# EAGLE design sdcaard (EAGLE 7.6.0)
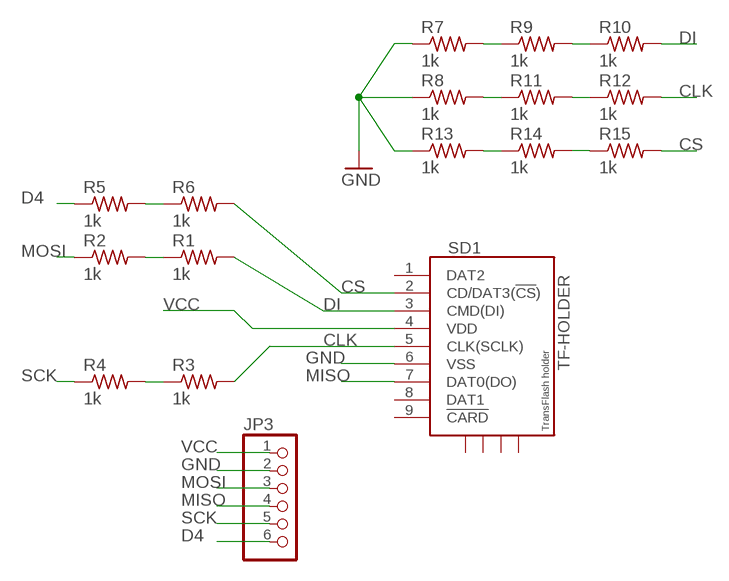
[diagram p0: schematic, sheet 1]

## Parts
JP3  PINHD-1X6  [1X06]
R1  1k  RES-US1206FAB  [R1206FAB]
R2  1k  RES-US1206FAB  [R1206FAB]
R3  1k  RES-US1206FAB  [R1206FAB]
R4  1k  RES-US1206FAB  [R1206FAB]
R5  1k  RES-US1206FAB  [R1206FAB]
R6  1k  RES-US1206FAB  [R1206FAB]
R7  1k  RES-US1206FAB  [R1206FAB]
R8  1k  RES-US1206FAB  [R1206FAB]
R9  1k  RES-US1206FAB  [R1206FAB]
R10  1k  RES-US1206FAB  [R1206FAB]
R11  1k  RES-US1206FAB  [R1206FAB]
R12  1k  RES-US1206FAB  [R1206FAB]
R13  1k  RES-US1206FAB  [R1206FAB]
R14  1k  RES-US1206FAB  [R1206FAB]
R15  1k  RES-US1206FAB  [R1206FAB]
SD1  TF-HOLDER  [TF-PULL]

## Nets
CLK: R3.2 R12.2 SD1.5(CLK(SCLK))
CS: R6.2 R15.2 SD1.2(CD/DAT3(!CS!))
D4: JP3.6 R5.1
DI: R1.2 R10.2 SD1.3(CMD(DI))
GND: JP3.2 R7.1 R8.1 R13.1 SD1.6(VSS)
MISO: JP3.4 SD1.7(DAT0(DO))
MOSI: JP3.3 R2.1
N$5: R1.1 R2.2
N$6: R5.2 R6.1
N$7: R3.1 R4.2
N$8: R13.2 R14.1
N$9: R14.2 R15.1
N$10: R8.2 R11.1
N$11: R7.2 R9.1
N$12: R9.2 R10.1
N$13: R11.2 R12.1
SCK: JP3.5 R4.1
VCC: JP3.1 SD1.4(VDD)
Unconnected: SD1.1(DAT2) SD1.8(DAT1) SD1.9(!CARD) SD1.S1 SD1.S2 SD1.S3 SD1.S4

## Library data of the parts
JP3 = pinhead:PINHD-1X6: PIN HEADER
R1-R15 = fab:RES-US: Resistor (US Symbol)
SD1 = sd-mmc:TF-HOLDER: TF / Micro SD socket is PUSH-PUSH type, the card can be pushed into and auto locked and pushed out by simply press the card. Surface Mounting type.

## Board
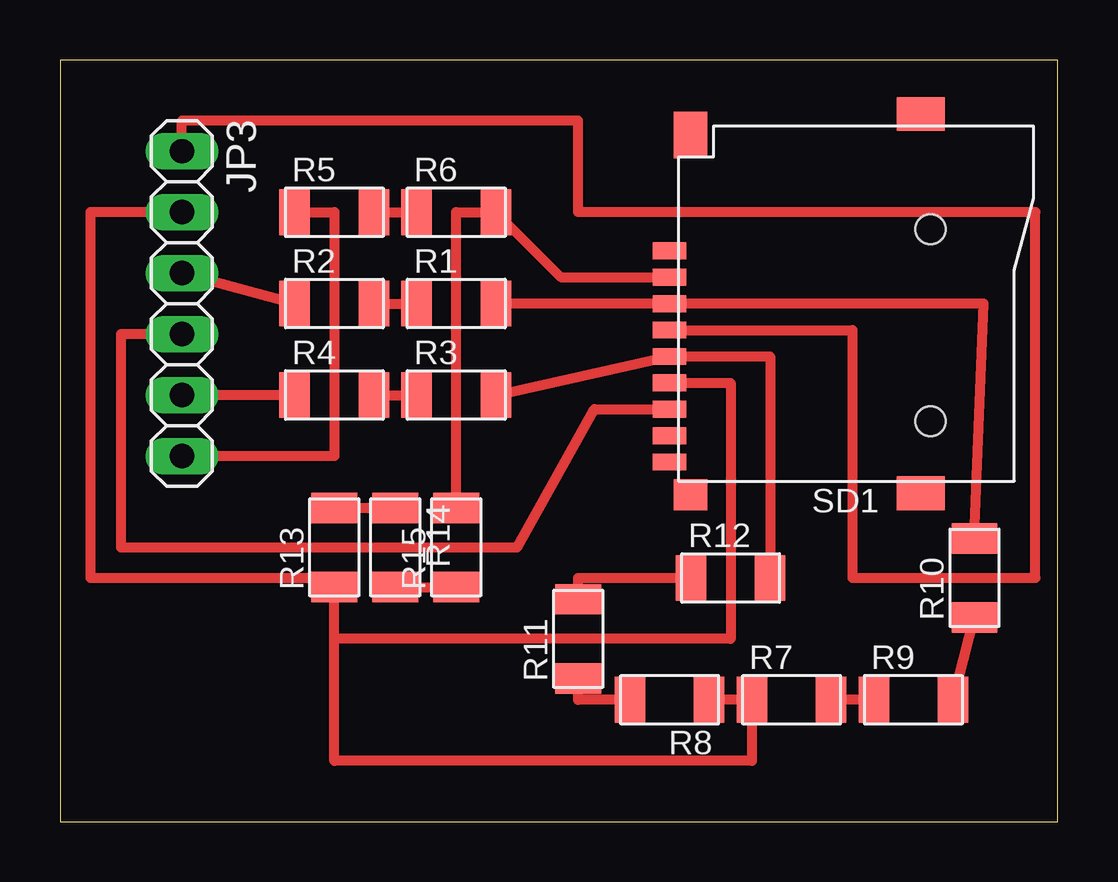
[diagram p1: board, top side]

Size 41.58 x 31.74 mm. Coordinates in mm from the lower left corner, seen from the top.
Outline: 0,0 41.58,0 41.58,31.74 0,31.74 0,0
Copper layers (1*16): Top 0.035mm / dielectric 1.5mm / Bottom 0.035mm
Design rules "default": minimum track width 10mil, minimum drill 24mil, track to track 8mil, track to pad 8mil, pad to pad 8mil, via to via 8mil, smd to smd 8mil, copper to edge 40mil, drill to drill 8mil, minimum pad ring 10mil, minimum via ring 8mil, stop-mask expansion 4mil, vias tented up to drill 0mil, thermal gap 10mil

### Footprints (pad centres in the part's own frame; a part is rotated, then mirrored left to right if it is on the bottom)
1X06 = drill 1.016 long: 1 -6.35,0; 2 -3.81,0; 3 -1.27,0; 4 1.27,0; 5 3.81,0; 6 6.35,0
R1206FAB = smd 1.27 x 1.905: 1 -1.651,0; 2 1.651,0
TF-PULL = smd 0.7 x 1.4: 1 -2.2,-7.62; 2 -1.1,-7.62; 3 0,-7.62; 4 1.1,-7.62; 5 2.2,-7.62; 6 3.3,-7.62; 7 4.4,-7.62; 8 5.5,-7.62; 9 6.6,-7.62 | smd 1.4 x 2: S1 -7.9,2.85; S2 7.9,2.85 | smd 1.28 x 1.4: S3 7.96,-6.75 | smd 1.95 x 1.4: S4 -7.025,-6.75 | hole 1.25: -3.1,3.25; 4.9,3.25

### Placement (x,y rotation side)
JP3  5.08,21.59 270 top
R1  16.51,21.59 0 top
R2  11.43,21.59 0 top
R3  16.51,17.78 0 top
R4  11.43,17.78 0 top
R5  11.43,25.4 0 top
R6  16.51,25.4 0 top
R7  30.48,5.08 0 top
R8  25.4,5.08 180 top
R9  35.56,5.08 0 top
R10  38.1,10.16 90 top
R11  21.59,7.62 90 top
R12  27.94,10.16 0 top
R13  11.43,11.43 90 top
R14  13.97,11.43 270 top
R15  16.51,11.43 90 top
SD1  33.02,21.59 270 top

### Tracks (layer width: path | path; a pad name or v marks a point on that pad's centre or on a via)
CLK
  Top 0.406: R3.2 SD1.5 29.59,19.39 R12.2
CS
  Top 0.406: SD1.2 20.87,22.69 R6.2 16.51,25.4 R15.2
D4
  Top 0.406: R5.1 11.43,25.4 11.43,15.24 JP3.6
DI
  Top 0.406: R1.2 SD1.3 38.48,21.59 R10.2
GND
  Top 0.406: JP3.2 1.27,25.4 1.27,10.16 11.43,10.16 R13.1 | R8.1 R7.1 28.83,2.54 11.43,2.54 R13.1 | SD1.6 27.94,18.29 27.94,7.62 11.43,7.62 R13.1
MISO
  Top 0.406: JP3.4 2.54,20.32 2.54,11.43 19.05,11.43 22.27,17.19 SD1.7
MOSI
  Top 0.406: R2.1 JP3.3
N$5
  Top 0.406: R2.2 R1.1
N$6
  Top 0.406: R5.2 R6.1
N$7
  Top 0.406: R4.2 R3.1
N$8
  Top 0.406: R13.2 R14.1
N$9
  Top 0.406: R14.2 R15.1
N$10
  Top 0.406: R8.2 21.59,5.08 R11.1
N$11
  Top 0.406: R9.1 R7.2
N$12
  Top 0.406: R9.2 R10.1
N$13
  Top 0.406: R11.2 21.59,10.16 R12.1
SCK
  Top 0.406: R4.1 JP3.5
VCC
  Top 0.406: JP3.1 5.08,29.21 21.59,29.21 21.59,25.4 40.64,25.4 40.64,10.16 33.02,10.16 33.02,20.49 SD1.4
